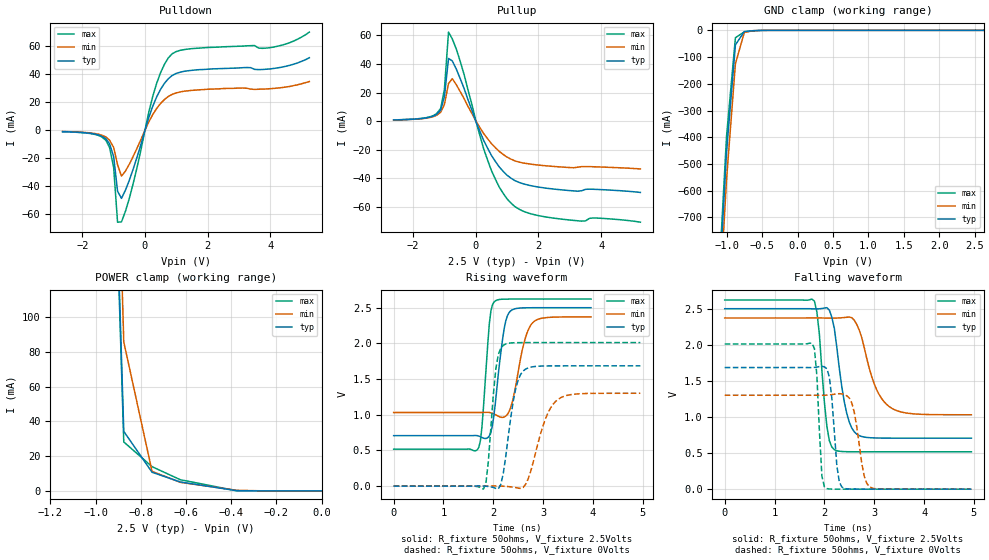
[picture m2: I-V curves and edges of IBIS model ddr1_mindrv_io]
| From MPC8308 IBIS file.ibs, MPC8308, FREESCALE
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[Model]   ddr1_mindrv_io   |
Model_type   I/O
Vinl = 1.22
Vinh = 1.28
Vmeas = 1.25
Cref = 1E-11
Rref = 50
Vref = 1.25
| variable   typ   min   max
C_comp   1.17p   1.10p   1.23p
[Model Spec]
| subparameter   typ   min   max
S_overshoot_high  3.300   3.135   3.465
S_overshoot_low   -200.00m  -100.00m  -300.00m
D_overshoot_high  4.000   4.000   4.000
D_overshoot_low   -1.000   -1.000   -1.000
D_overshoot_time  1.000n   1.000n   1.000n
| variable   typ   min   max
[Temperature Range]   25.0   -40.0   125.0
| variable   typ   min   max
[Pullup Reference]   2.500V   2.375V   2.625V
| variable   typ   min   max
[Pulldown Reference]   0.000V   0.000V   0.000V
| variable   typ   min   max
[POWER_Clamp_Reference]   2.500V   2.375V   2.625V
| variable   typ   min   max
[GND_Clamp_Reference]   0.000V   0.000V   0.000V
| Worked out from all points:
|   slope of the pulldown table from 0 to 0.375 V, typ, clamps not added: 15.7 ohm
|   slope of the pullup table from 0 to 0.375 V, typ, clamps not added: 20 ohm
|   GND clamp passes 1 mA (typ) near -0.59 V on its own axis
|   POWER clamp passes 1 mA (typ) near -0.42 V on its own axis
|   rising waveform, R_fixture 50ohms, V_fixture 2.5Volts: 20-80 % time 179ps typ, 237ps min, 128ps max; typ from 0.707 V to 2.5 V
|   rising waveform, R_fixture 50ohms, V_fixture 0Volts: 20-80 % time 211ps typ, 337ps min, 139ps max; typ from 0 V to 1.69 V
|   falling waveform, R_fixture 50ohms, V_fixture 2.5Volts: 20-80 % time 228ps typ, 361ps min, 149ps max; typ from 2.5 V to 0.707 V
|   falling waveform, R_fixture 50ohms, V_fixture 0Volts: 20-80 % time 114ps typ, 172ps min, 87.9ps max; typ from 1.69 V to 0 V
[Pulldown]
| pulldown in the table = pulldown subtract gnd_clamp
|Voltage   I(typ)   I(min)   I(max)
-2.63V    -970uA     -880uA     -1.02mA
-1.25V    -5.98mA    -4.72mA    -7.04mA
-1.13V    -9.64mA    -7.06mA    -12.3mA
-1V       -18.8mA    -12.2mA    -26.5mA
-875mV    -43.5mA    -24.6mA    -65.6mA
-750mV    -48.6mA    -32.7mA    -65.4mA
-375mV    -27.6mA    -18.6mA    -37.9mA
125mV     9.32mA     6.07mA     13.2mA
375mV     23.9mA     15.6mA     33.6mA
875mV     39.2mA     25.7mA     54.7mA
4V        43.8mA     29.7mA     59mA
5.25V     51.8mA     34.8mA     70.1mA
[Pullup]
| pullup in the table = pullup subtract power_clamp
|Voltage   I(typ)   I(min)   I(max)
-2.62V    860.9uA    825uA      897.4uA
-1.5V     2.637mA    2.394mA    2.836mA
-1.12V    7.69mA     6.205mA    8.854mA
-1V       17.29mA    11.7mA     22.48mA
-870mV    43.76mA    26.27mA    62.19mA
-750mV    42.11mA    29.67mA    57.48mA
-370mV    22.68mA    15.67mA    32.33mA
380mV     -18.97mA   -12.34mA   -27.36mA
750mV     -31.99mA   -21.14mA   -46.07mA
1.13V     -39.89mA   -26.58mA   -57.33mA
2.38V     -47.11mA   -31.41mA   -67.34mA
5.25V     -49.75mA   -33.34mA   -70.51mA
[GND_clamp]
|Voltage   I(typ)   I(min)   I(max)
-2.625V   -9.497A    -9.494A    -9.517A
-1.125V   -1.057A    -1.145A    -1.012A
-1V       -454.7mA   -557.3mA   -396.5mA
-875mV    -54.6mA    -124.7mA   -27.53mA
-750mV    -4.635mA   -8.012mA   -5.794mA
-625mV    -1.367mA   -1.259mA   -1.854mA
-500mV    -191.1uA   -225.6uA   -219.2uA
2.625V    45.37nA    27.37uA    16.83pA
[POWER_clamp]
|Voltage   I(typ)   I(min)   I(max)
-2.375V   9.526A     9.538A     9.599A
-1.125V   1.078A     1.196A     1.069A
-875mV    34.28mA    85.75mA    28.2mA
-750mV    10.75mA    11.29mA    13.96mA
-625mV    5.151mA    4.938mA    6.448mA
-375mV    135.8uA    350uA      84.92uA
0V        255.3pA    14.06nA    16.83pA
[Ramp]
|Voltage   I(typ)   I(min)   I(max)
dV/dt_f   1.08/227.016p 0.81/362.218p 1.27/146.040p
dV/dt_r   1.03/213.645p 0.80/343.259p 1.23/140.661p
R_load=50ohms
| R_load was connected to ground for Ramp_up test and power for Ramp_dn test
[Rising_Waveform]
R_fixture=50ohms
V_fixture=2.5Volts
V_fixture_min=2.375Volts
V_fixture_max=2.625Volts
|C_fixture=1E-15f
|L_fixture=1E-15h
|C_dut=1E-15fh
|R_dut=0.001ohm
|L_dut=1E-12h
|time   V(typ)   V(min)   V(max)
0s        707mV      1.031V     518mV
1.68ns    707mV      1.031V     510mV
1.77ns    682mV      1.031V     817mV
1.92ns    705mV      1.032V     2.28V
2.04ns    1.16V      1.002V     2.596V
2.22ns    2.217V     968mV      2.62V
2.34ns    2.451V     1.086V     2.621V
2.61ns    2.498V     1.992V     2.621V
2.79ns    2.5V       2.29V      2.621V
3.96ns    2.5V       2.372V     2.621V
[Rising_Waveform]
R_fixture=50ohms
V_fixture=0Volts
|C_fixture=1E-15f
|L_fixture=1E-15h
|C_dut=1E-15fh
|R_dut=0.001ohm
|L_dut=1E-12h
|time   V(typ)   V(min)   V(max)
0s        9.109nV    808.2nV    116pV
1.8ns     1.382mV    -203uV     -42.75mV
1.9ns     -5.107mV   1.028mV    346.3mV
2.05ns    -31.82mV   2.241mV    1.642V
2.2ns     180.2mV    -1.528mV   1.973V
2.4ns     1.193V     -14.78mV   2.008V
2.6ns     1.614V     -17.4mV    2.011V
3.05ns    1.684V     949.6mV    2.011V
3.3ns     1.685V     1.216V     2.011V
4.95ns    1.685V     1.301V     2.011V
[Falling_Waveform]
R_fixture=50ohms
V_fixture=2.5Volts
V_fixture_min=2.375Volts
V_fixture_max=2.625Volts
|C_fixture=1E-15f
|L_fixture=1E-15h
|C_dut=1E-15fh
|R_dut=0.001ohm
|L_dut=1E-12h
|time   V(typ)   V(min)   V(max)
0s        2.5V       2.372V     2.621V
1.8ns     2.498V     2.372V     2.605V
1.9ns     2.499V     2.372V     2.145V
2.05ns    2.515V     2.37V      872.2mV
2.2ns     2.226V     2.37V      547mV
2.4ns     1.208V     2.378V     520.2mV
2.65ns    761.6mV    2.282V     518mV
3ns       709.9mV    1.459V     517.9mV
3.3ns     707mV      1.145V     517.9mV
4.95ns    706.7mV    1.031V     517.9mV
[Falling_Waveform]
R_fixture=50ohms
V_fixture=0Volts
|C_fixture=1E-15f
|L_fixture=1E-15h
|C_dut=1E-15fh
|R_dut=0.001ohm
|L_dut=1E-12h
|time   V(typ)   V(min)   V(max)
0s        1.685V     1.301V     2.011V
1.75ns    1.684V     1.301V     2.022V
1.85ns    1.692V     1.301V     1.569V
1.95ns    1.701V     1.3V       183.1mV
2.05ns    1.669V     1.302V     7.974mV
2.25ns    325.9mV    1.32V      299.8uV
2.35ns    30.53mV    1.32V      86.15uV
2.55ns    1.32mV     1.196V     7.41uV
2.9ns     70.43uV    36.76mV    -212.8nV
4.95ns    -20.77nV   611.4nV    -12.58nV
